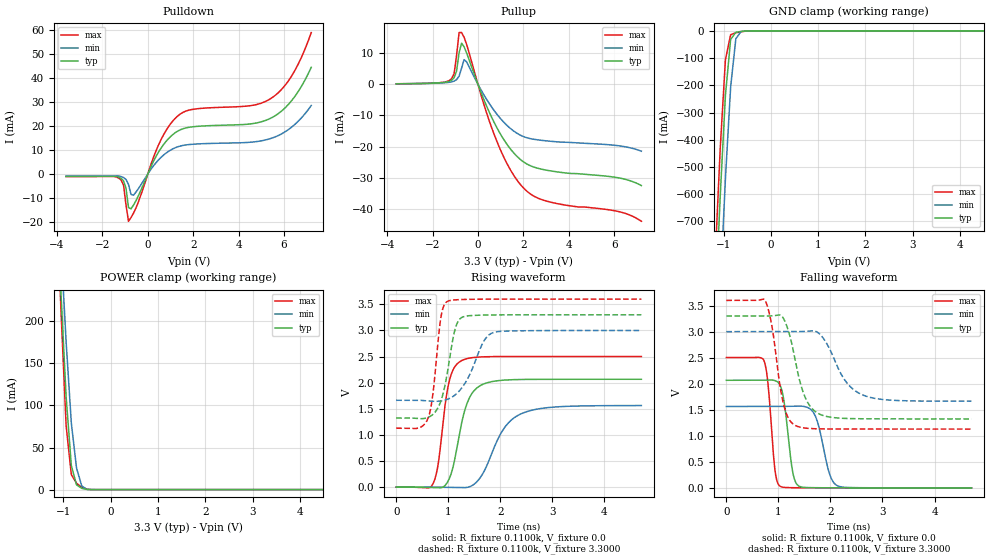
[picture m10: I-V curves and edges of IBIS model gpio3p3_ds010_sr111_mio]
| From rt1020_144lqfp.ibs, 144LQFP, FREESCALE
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[Model] gpio3p3_ds010_sr111_mio
|   Model gpio3p3_ds010_sr111_mio
| This model was characterised for following simulation conditions:
| External (pad) voltage:
|   - Typ: 3.3V,   - Min: 3.0V,   - Max: 3.6V
| Library cells for typ/min/max conditions are connected as defined below:
|  pad - External Pad
|  ipp_do - Core Input
|  ipp_obe - Output Buffer Enable
|  esd_boost - ovdd
|  ipp_dse0 - vssi
|  ipp_dse1 - vddi
|  ipp_dse2 - vssi
|  ipp_fsel0 - vddi
|  ipp_fsel1 - vddi
|  ipp_ina - ipp_ina
|  ipp_ind - ipp_ind
|  ipp_pwr_stable - vddi
|  ipp_sre - vddi
|  ovdd - ovdd
|  ovss - ovss
|  vddi - vddi
|  vssi - vssi
| All other pins connected to ground
Model_type I/O
Polarity   Non-Inverting
Enable   Active-High
Vinl =   0.9900V
Vinh =   2.3100V
Vmeas =  1.6500V
Cref =   0.0F
Rref =   0.1100k
Vref =   1.6500V
C_comp   1.2179pF   1.1833pF   1.2636pF
|C_comp_pullup   0.6043pF   0.6190pF   0.5909pF
|C_comp_pulldown   0.5474pF   0.5788pF   0.5258pF
[Model Spec]
| variable   typ   min   max
Vinh   2.3100V   2.1000V   2.5200V
Vinl   0.9900V   0.9000V   1.0800V
S_overshoot_high   3.3000V   3.0000V   3.6000V
S_overshoot_low   0.0V   0.0V   0.0V
Vmeas   1.6500V   1.5000V   1.8000V
Vref   1.6500V   1.5000V   1.8000V
Cref   0.0F   0.0F   0.0F
Rref   0.1100k   0.1100k   0.1100k
[Temperature Range]   25.0000   0.1050k   -20.0000
[Voltage Range]   3.3000V   3.0000V   3.6000V
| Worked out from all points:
|   slope of the pulldown table from 0 to 0.495 V, typ, clamps not added: 52.1 ohm
|   slope of the pullup table from 0 to 0.495 V, typ, clamps not added: 55.8 ohm
|   GND clamp passes 1 mA (typ) near -0.54 V on its own axis
|   POWER clamp passes 1 mA (typ) near -0.57 V on its own axis
|   rising waveform, R_fixture 0.1100k, V_fixture 0.0: 20-80 % time 282ps typ, 482ps min, 197ps max; typ from 0 V to 2.07 V
|   rising waveform, R_fixture 0.1100k, V_fixture 3.3000: 20-80 % time 222ps typ, 367ps min, 156ps max; typ from 1.32 V to 3.3 V
|   falling waveform, R_fixture 0.1100k, V_fixture 0.0: 20-80 % time 147ps typ, 213ps min, 117ps max; typ from 2.07 V to 0 V
|   falling waveform, R_fixture 0.1100k, V_fixture 3.3000: 20-80 % time 299ps typ, 443ps min, 219ps max; typ from 3.3 V to 1.32 V
[Pulldown]
|Voltage   I(typ)   I(min)   I(max)
-3.6V     -1.02mA    -860uA     -1.08mA
-1.29V    -1.294mA   -833uA     -1.653mA
-1.07V    -2.852mA   -1.461mA   -4.561mA
-960mV    -5.973mA   -2.272mA   -13mA
-850mV    -14.01mA   -4.368mA   -19.77mA
-630mV    -13.01mA   -8.848mA   -16.37mA
470mV     9.13mA     5.875mA    12.09mA
1.24V     17.47mA    11.09mA    23.58mA
1.9V      19.64mA    12.38mA    26.89mA
5.42V     23.36mA    14.86mA    31.56mA
6.3V      30.26mA    19.33mA    40.44mA
7.2V      44.59mA    28.62mA    59.13mA
[Pullup]
|Voltage   I(typ)   I(min)   I(max)
-3.6V     150uA      130uA      150uA
-1.16V    1.269mA    750uA      1.777mA
-1.05V    2.063mA    994uA      3.366mA
-940mV    4.231mA    1.48mA     9.243mA
-830mV    10.07mA    2.574mA    16.54mA
-720mV    13.14mA    5.17mA     16.54mA
-610mV    11.98mA    7.864mA    15.04mA
-500mV    10.04mA    7.165mA    12.8mA
820mV     -13.71mA   -9.439mA   -18.03mA
2.03V     -24.96mA   -16.82mA   -33.37mA
3.02V     -27.5mA    -18.13mA   -37.4mA
7.2V      -32.44mA   -21.43mA   -43.87mA
[GND_clamp]
|Voltage   I(typ)   I(min)   I(max)
-3.6V     -10.99A    -11.14A    -10.93A
-1.18V    -1.033A    -1.378A    -850.8mA
-1.07V    -607mA     -947.1mA   -431.4mA
-960mV    -236.8mA   -543mA     -106.4mA
-850mV    -31.63mA   -206.7mA   -14.18mA
-740mV    -5.424mA   -29mA      -7.092mA
-630mV    -2.275mA   -2.653mA   -3.283mA
-410mV    -62.05uA   -83.52uA   -82.04uA
7.2V      0A         0A         0A
[POWER_clamp]
|Voltage   I(typ)   I(min)   I(max)
-3.6V     3.491A     3.319A     3.949A
-1.16V    368.2mA    410.8mA    372.9mA
-1.05V    234.5mA    290.2mA    214.3mA
-940mV    110.2mA    175.6mA    75.85mA
-830mV    28.53mA    79.02mA    17.73mA
-720mV    5.671mA    25.66mA    7.515mA
-610mV    1.49mA     4.301mA    2.636mA
-500mV    198.2uA    300.8uA    424.4uA
-390mV    9.667uA    18.86uA    16.14uA
7.2V      0A         0A         0A
[Ramp]
| variable   typ   min   max
dV/dt_r  1.2395/0.2815n   0.9376/0.4815n   1.5013/0.1969n
dV/dt_f  1.1854/0.2987n   0.8015/0.4428n   1.4826/0.2191n
R_load = 0.1100k
[Rising Waveform]
R_fixture= 0.1100k
V_fixture= 0.0
V_fixture_min= 0.0
V_fixture_max= 0.0
|time   V(typ)   V(min)   V(max)
0s        8.464nV    7.651nV    89.62nV
703.3ps   -5.512mV   184uV      59.36mV
801.8ps   -10.14mV   -587.6uV   413.7mV
1.011ns   144.6mV    -2.967mV   1.997V
1.254ns   1.219V     -8.376mV   2.422V
1.378ns   1.649V     -551.9uV   2.465V
1.573ns   1.917V     129.3mV    2.491V
2.062ns   2.049V     1.113V     2.501V
2.377ns   2.061V     1.394V     2.502V
4.71ns    2.066V     1.563V     2.502V
[Rising Waveform]
R_fixture= 0.1100k
V_fixture= 3.3000
V_fixture_min= 3.0000
V_fixture_max= 3.6000
|time   V(typ)   V(min)   V(max)
0s        1.324V     1.664V     1.129V
606.6ps   1.333V     1.652V     1.308V
708.3ps   1.396V     1.645V     1.812V
854.6ps   1.639V     1.65V      3.227V
991.7ps   2.247V     1.685V     3.56V
1.119ns   2.975V     1.756V     3.585V
1.22ns    3.216V     1.851V     3.591V
1.675ns   3.294V     2.78V      3.599V
1.861ns   3.297V     2.958V     3.599V
4.71ns    3.3V       3V         3.6V
[Falling Waveform]
R_fixture= 0.1100k
V_fixture= 0.0
V_fixture_min= 0.0
V_fixture_max= 0.0
|time   V(typ)   V(min)   V(max)
0s        2.066V     1.563V     2.502V
725.8ps   2.068V     1.563V     2.438V
798.4ps   2.07V      1.563V     2.02V
934.2ps   2.06V      1.563V     343.5mV
1.037ns   1.961V     1.564V     28.97mV
1.27ns    333.6mV    1.568V     3.04mV
1.404ns   29.09mV    1.571V     1.567mV
1.694ns   2.93mV     1.413V     573.9uV
2.148ns   582uV      34.42mV    258.7uV
4.71ns    16.1uV     75.36uV    11.57uV
[Falling Waveform]
R_fixture= 0.1100k
V_fixture= 3.3000
V_fixture_min= 3.0000
V_fixture_max= 3.6000
|time   V(typ)   V(min)   V(max)
0s        3.3V       3V         3.6V
755.3ps   3.299V     3V         3.579V
880.5ps   3.303V     3V         3.08V
1.089ns   3.268V     3V         1.649V
1.325ns   2.442V     3V         1.198V
1.535ns   1.692V     3.006V     1.146V
1.867ns   1.386V     2.868V     1.132V
2.269ns   1.334V     2.08V      1.129V
2.621ns   1.327V     1.784V     1.129V
4.71ns    1.324V     1.664V     1.129V
